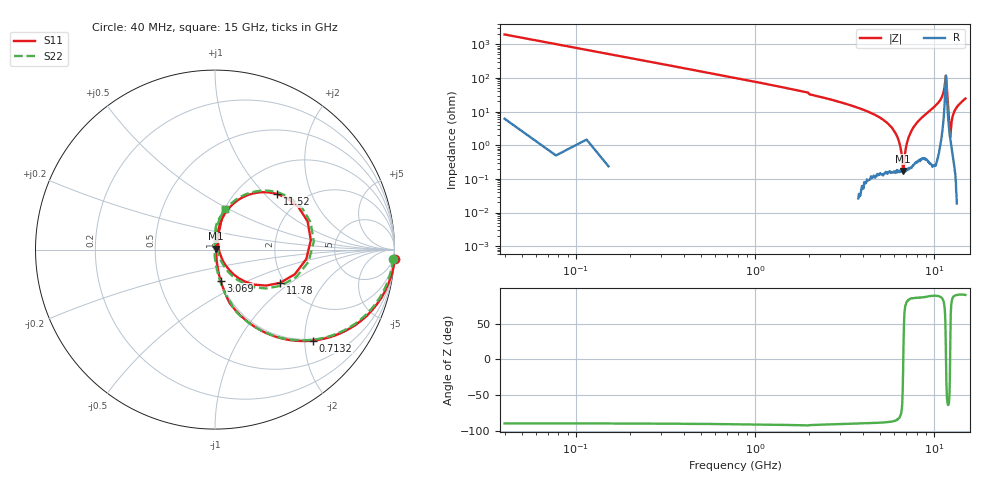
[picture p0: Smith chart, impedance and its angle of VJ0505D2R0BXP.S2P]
! VJ0505D2R0BXP
! MLCC placed on 25 mil thick microstrip substrate in series configuraton.
! DATE 06/29/2018  07:32
! CORRECTED  DATA
# GHz  S  MA  R  50.00
!  FREQ  S11M  S11A  S21M  S21A  S12M  S12A  S22M  S22A
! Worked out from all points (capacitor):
!   401 points, 40 MHz to 15 GHz, reference 50 ohm
!   read as one part in series: C = 2.03 pF near 114.8 MHz
!   lowest |Z| = 172 mohm at 6.735 GHz (marker M1)
!   series resonance near 6.748 GHz, so ESL is about 270 pH
!   S11 on the Smith chart (normalised r, x): 40 MHz: -2, -39; 713.2 MHz: 0.96, -2.19; 3.069 GHz: 1.00, -0.36; 11.52 GHz: 1.49, +1.18; 11.78 GHz: 1.89, -0.84; 15 GHz: 1.00, +0.47
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0.04  1.002 -2.9  0.05105 86.9  0.05133 87.4  0.9946 -2.9
0.2644  0.9522 -18.6  0.3201 71.5  0.3202 71.5  0.9444 -18.6
0.7132  0.7452 -42.9  0.6811 48.0  0.6817 48.0  0.7399 -42.8
1.4238  0.475 -63.4  0.8962 28.5  0.8968 28.5  0.474 -63.5
2.5458  0.2331 -77.5  0.9772 13.8  0.9776 13.9  0.2342 -77.6
3.0694  0.1767 -79.6  0.9855 10.7  0.986 10.7  0.1798 -80.8
5.0516  0.05923 -81.2  0.9965 3.9  0.9967 4.0  0.05855 -88.9
6.024  0.02048 -69.4  0.9978 1.8  0.9983 1.8  0.01993 -98.4
6.585  0.006134 1.7  0.9975 0.6  0.9982 0.7  0.003818 -178.1
6.7346  0.008226 41.3  0.9977 0.3  0.9983 0.4  0.00625 125.2
7.0712  0.01804 69.0  0.9972 -0.3  0.9979 -0.3  0.01712 101.2
7.52  0.03343 77.2  0.9965 -1.3  0.9972 -1.3  0.03298 94.2
10.0258  0.1374 79.2  0.9867 -7.6  0.9877 -7.6  0.1406 83.9
11.1104  0.2605 69.7  0.943 -15.1  0.9437 -15.1  0.2684 71.1
11.5218  0.4643 42.0  0.7204 -25.7  0.721 -25.7  0.4774 41.7
11.6714  0.5366 5.7  0.4609 -6.1  0.4608 -6.1  0.5521 4.6
11.7836  0.4073 -27.1  0.6638 16.9  0.6641 16.9  0.4186 -28.8
12.0828  0.09445 -56.0  0.9535 4.8  0.9542 4.8  0.09467 -61.7
12.3072  0.02287 -7.9  0.9817 0.1  0.9824 0.1  0.01206 -18.4
12.5316  0.04431 67.2  0.9894 -2.5  0.99 -2.5  0.04271 85.6
13.1674  0.111 77.3  0.9911 -6.7  0.9916 -6.7  0.114 88.6
15  0.2309 76.6  0.9713 -14.2  0.9718 -14.2  0.232 75.8
